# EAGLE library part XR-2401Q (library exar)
MICROCONTROLLER
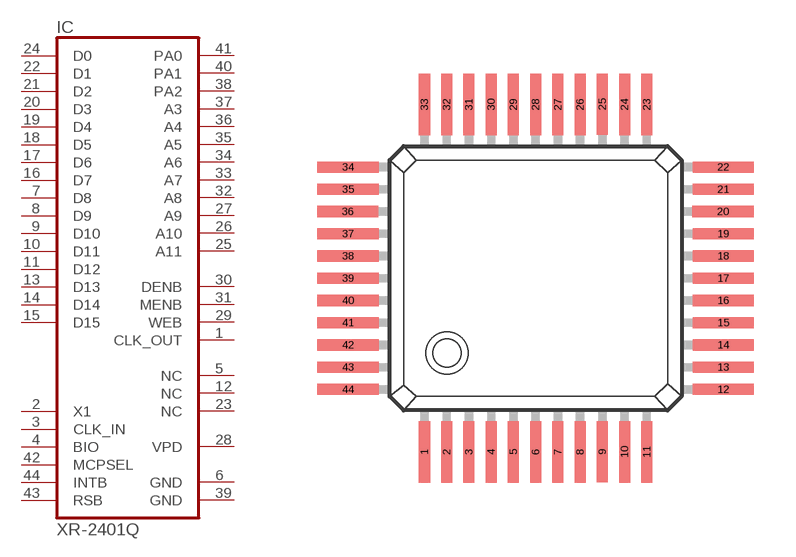
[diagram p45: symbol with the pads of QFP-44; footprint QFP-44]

Designator prefix IC

## XR-2401Q (OC_FARNELL: unknown; OC_NEWARK: unknown)  [QFP-44]
1  CLK_OUT  out
2  X1  in
3  CLK_IN  in
4  BIO  in
5  NC  nc
6  GND  pwr
7  D8
8  D9
9  D10
10  D11
11  D12
12  NC  nc
13  D13
14  D14
15  D15
16  D7
17  D6
18  D5
19  D4
20  D3
21  D2
22  D1
23  NC  nc
24  D0
25  A11  out
26  A10  out
27  A9  out
28  VPD  pwr
29  WEB  out
30  DENB  out
31  MENB  out
32  A8  out
33  A7  out
34  A6  out
35  A5  out
36  A4  out
37  A3  out
38  PA2  out
39  GND  pwr
40  PA1  out
41  PA0  out
42  MCPSEL  in
43  RSB  in
44  INTB  in

## Footprint QFP-44 (pad centres in mm)
Quad Flat Package
smd 0.4 x 2.2: 1 -4,-6.25; 2 -3.2,-6.25; 3 -2.4,-6.25; 4 -1.6,-6.25; 5 -0.8,-6.25; 6 0,-6.25; 7 0.8,-6.25; 8 1.6,-6.25; 9 2.4,-6.24; 10 3.2,-6.25; 11 4,-6.25; 23 4,6.25; 24 3.2,6.25; 25 2.4,6.26; 26 1.6,6.25; 27 0.8,6.25; 28 0,6.25; 29 -0.8,6.25; 30 -1.6,6.25; 31 -2.4,6.25; 32 -3.2,6.25; 33 -4,6.25
smd 2.2 x 0.4: 12 6.75,-4; 13 6.75,-3.2; 14 6.75,-2.4; 15 6.75,-1.6; 16 6.75,-0.8; 17 6.75,0; 18 6.75,0.8; 19 6.75,1.6; 20 6.74,2.4; 21 6.75,3.2; 22 6.75,4; 34 -6.75,4; 35 -6.75,3.2; 36 -6.76,2.4; 37 -6.75,1.6; 38 -6.75,0.8; 39 -6.75,0; 40 -6.75,-0.8; 41 -6.75,-1.6; 42 -6.75,-2.4; 43 -6.75,-3.2; 44 -6.75,-4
